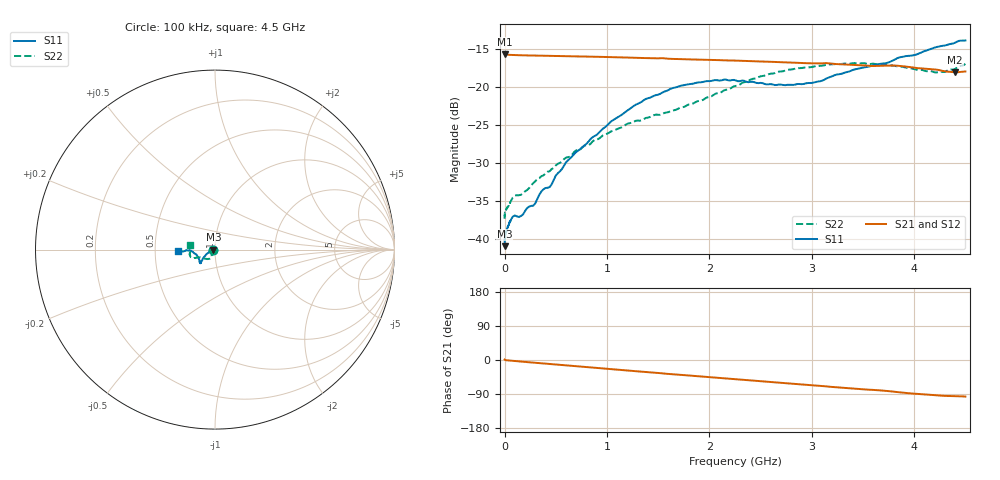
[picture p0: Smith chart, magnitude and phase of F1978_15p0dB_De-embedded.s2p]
! Integrated Device Technology
! Corporate Headquarters
! 6024 Silver Creek Valley Road
! San Jose, CA 95138  USA
! Phone:  1-408-284-8200
! Toll Free:  1-800-223-1366
! Webpage:  http://www.idt.com/
! Timing and RF Division
! 515 Groton Road, Suite 102
! Westford, MA 01886-6024
! Device:  F1978
! Description: 6-bit, 75 ohm, 0.5 dB Digital Step Attenuator
! Frequency:  5.0 MHz -  3.00 GHz
! Package:  4x4 mm QFN Plastic Package: 20 pin
! Ports:  2 RF, 11 DC
!  Pin  1  = D5 (16 dB)
!  Pin  2  = RF1  =  Port 1
!  Pin  3  = Serial Data In (DATA)
!  Pin  4  = Serial Clock (CLK)
!  Pin  5  = Serial Latch Enable (LE)
!  Pin  6  = VDD
!  Pin  7  = NC
!  Pin  8  = NC
!  Pin  9  = NC
!  Pin 10  = GND
!  Pin 11  = GND
!  Pin 12  = NC
!  Pin 13  = VMODE
!  Pin 14  = RF2  =  Port 2
!  Pin 15  = D4 (8 dB)
!  Pin 16  = D3 (4 dB)
!  Pin 17  = D2 (2 dB)
!  Pin 18  = NC
!  Pin 19  = D1 (1 dB)
!  Pin 20  = D0 (0.5 dB)
! State:  30
! Atten State:  15.0 dB
! Voltage:  +3.30 Volts
! Current:  0.594 mA
! Data:  The device was measured on a F1975 evaluation board which has
!  individual transmission lines to the RF pins.  Data was collected
!  using a calibrated network analyzer.  The evaluation board was
!  de-embedded using Automatic Fixture Removal (AFR).
!  The reference plane is the edge of the package pin.
! Misc:
!  Action Tracker AT0416
! Date Measured:  2018-02-08
! Date:  2018-03-26  MJV
! Note:
!  Integrated Device Technology supplies this data as a sample of measured
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# GHz S dB R 75
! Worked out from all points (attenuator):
!   291 points, 100 kHz to 4.5 GHz, reference 75 ohm
!   highest |S21| = -15.62 dB at 100 kHz (marker M1); lowest = -18.0 dB at 4.4 GHz (marker M2)
!   lowest |S11| = -41.0 dB at 100 kHz (marker M3), VSWR 1.02, Z = 73.7 + j0.0156 ohm
!   |S11| at or under -10 dB: start of sweep to end of sweep
!   |S22| runs from -37.4 to -16.8 dB; largest |S21 - S12| = 0.00021
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0.0001  -41.00 179.3  -15.62 1.2  -15.62 1.2  -37.37 -178.3
0.0009  -40.13 -175.8  -15.65 1.0  -15.64 1.1  -36.92 -177.7
0.005  -39.51 -175.5  -15.67 0.4  -15.67 0.4  -36.58 -175.4
0.08  -37.09 -168.9  -15.74 -2.2  -15.74 -2.2  -34.57 -162.0
0.16  -37.01 -166.1  -15.77 -4.1  -15.77 -4.1  -34.21 -147.2
0.22  -35.96 -166.8  -15.79 -5.5  -15.79 -5.5  -33.58 -140.3
0.28  -35.65 -165.1  -15.81 -6.9  -15.81 -6.9  -32.66 -136.9
0.36  -33.76 -165.7  -15.83 -8.7  -15.83 -8.7  -31.76 -128.7
0.44  -33.18 -163.0  -15.85 -10.5  -15.85 -10.5  -31.09 -123.3
0.6  -29.91 -161.2  -15.90 -14.2  -15.89 -14.2  -29.29 -119.7
0.76  -27.90 -155.4  -15.94 -17.8  -15.93 -17.8  -27.94 -118.0
1.26  -22.48 -145.7  -16.10 -29.1  -16.09 -29.1  -24.57 -120.3
1.52  -20.87 -141.0  -16.16 -34.7  -16.16 -34.7  -23.64 -127.7
1.88  -19.38 -137.3  -16.34 -42.6  -16.34 -42.6  -21.86 -142.9
2.26  -19.11 -138.8  -16.48 -50.8  -16.48 -50.8  -19.81 -154.2
2.58  -19.60 -148.2  -16.63 -57.7  -16.62 -57.7  -18.26 -157.5
3.02  -19.37 -165.3  -16.83 -66.8  -16.83 -66.8  -17.26 -161.2
3.42  -17.64 -176.3  -17.05 -75.7  -17.04 -75.7  -16.81 -167.6
3.76  -16.67 -177.9  -17.12 -82.3  -17.12 -82.3  -17.11 -174.4
4.2  -14.76 -176.6  -17.65 -92.8  -17.65 -92.8  -18.03 174.0
4.4  -14.11 -175.5  -18.02 -95.4  -18.01 -95.4  -17.58 171.0
4.5  -13.81 -177.4  -17.91 -96.6  -17.91 -96.6  -16.91 169.5
